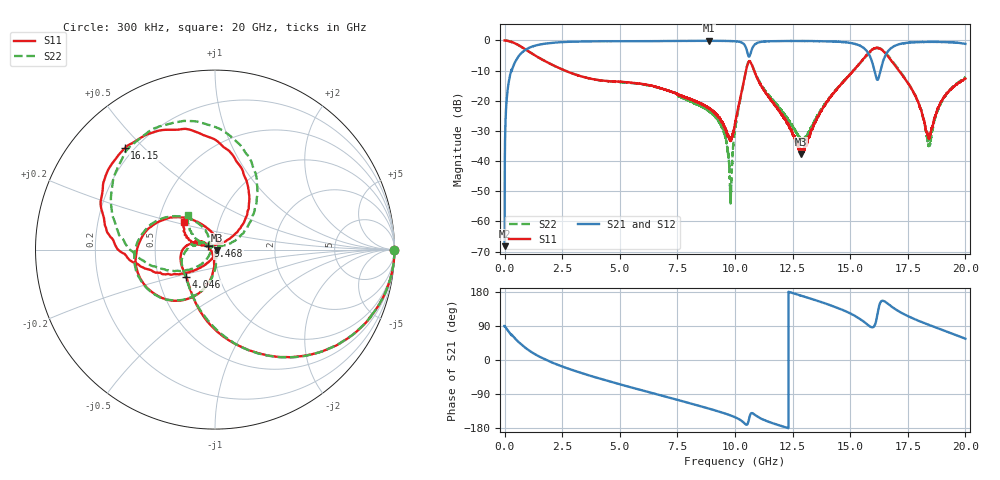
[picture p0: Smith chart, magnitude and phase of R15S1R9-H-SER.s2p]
!{R15S1R9}
!Johanson Technology Inc.
!www.johansontechnology.com
!Test Board Conditions:
!Substrate Type  RO4350B
!Substrate Thickness  20 mil
!Substrate Dk  3.66
!TL Type: GCPW
!TL Trace Width  34 mil
!TL Gap  10 mil
!Electrode orientation  Horizontal
!DUT TOPOLOGY	SERIES
!Mounting Pad LxW  26x52 mil
! Created Sat Feb  6 12:19:02 2021
# hz S ma R 50
! 2 Port Network Data from SP1.SP block
! freq  magS11  angS11  magS21  angS21  magS12  angS12  magS22  angS22
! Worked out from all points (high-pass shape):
!   20001 points, 300 kHz to 20 GHz, reference 50 ohm
!   highest |S21| = -0.12 dB at 8.878 GHz (marker M1); lowest = -68.2 dB at 300 kHz (marker M2)
!   |S21| within 3 dB of the highest: 904.7 MHz to 10.51 GHz (9.602 GHz wide, 168 % of centre); 10.73 GHz to 15.67 GHz (4.949 GHz wide, 37.5 % of centre)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
!   lowest |S11| = -37.6 dB at 12.87 GHz (marker M3), VSWR 1.03, Z = 51.3 - j0.353 ohm
!   |S11| at or under -10 dB: 2.623 GHz to 10.48 GHz (7.855 GHz wide, 120 % of centre); 10.83 GHz to 15.13 GHz (4.307 GHz wide, 33.2 % of centre); 17.12 GHz to end of sweep
!   |S22| runs from -54.0 to 0.0 dB; largest |S21 - S12| = 0.021
!   S11 on the Smith chart (normalised r, x): 300 kHz: open; 4.046 GHz: 0.70, -0.22; 9.468 GHz: 0.93, +0.03; 16.15 GHz: 0.16, +0.44; 20 GHz: 0.68, +0.22
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300000  1 -0.2  0.0003894 89.7  0.0002232 96.0  0.9969 -0.2
1.273e8  0.9886 -10.5  0.1472 79.2  0.148 79.2  0.9874 -10.5
4.713e8  0.8891 -33.8  0.4511 55.8  0.4524 55.9  0.8886 -33.9
1.5893e9  0.4924 -83.6  0.8628 6.4  0.8643 6.4  0.4916 -83.1
3.3343e9  0.2537 -123.9  0.961 -34.3  0.9607 -34.3  0.2546 -124.5
4.0463e9  0.221 -136.1  0.9691 -47.6  0.9685 -47.5  0.2212 -138.8
6.6673e9  0.1666 174.0  0.9754 -91.4  0.9763 -91.4  0.165 -176.4
8.8783e9  0.07517 147.2  0.9863 -128.6  0.984 -128.5  0.06747 143.2
9.4683e9  0.04252 154.2  0.9823 -139.2  0.9825 -139.4  0.03499 126.1
9.7963e9  0.02271 -155.2  0.977 -146.0  0.9787 -146.0  0.002608 166.0
1.00003e10  0.04215 -102.9  0.9702 -151.0  0.9701 -150.9  0.03238 -80.9
1.06403e10  0.4477 -169.9  0.5536 -148.3  0.5554 -148.5  0.4544 -171.5
1.13133e10  0.1386 113.3  0.9626 -159.6  0.9627 -159.7  0.1463 119.1
1.28743e10  0.01321 -15.1  0.9791 169.6  0.978 169.7  0.02349 165.8
1.33343e10  0.0332 -91.4  0.9772 160.9  0.9774 161.0  0.03799 -140.2
1.53253e10  0.3777 -162.6  0.8479 112.0  0.8476 111.9  0.3814 -168.0
1.61513e10  0.7583 131.6  0.2293 110.4  0.2299 110.6  0.7492 121.8
1.66673e10  0.5278 78.5  0.6817 146.9  0.6783 148.4  0.548 69.7
1.78773e10  0.1091 36.9  0.9365 105.8  0.9353 105.4  0.111 23.8
1.84193e10  0.02341 106.5  0.9456 92.7  0.9443 92.6  0.01781 91.4
1.90013e10  0.1031 162.4  0.9419 79.3  0.9418 79.3  0.1008 152.6
2e10  0.2325 138.1  0.8774 56.2  0.8709 56.1  0.2458 126.6
